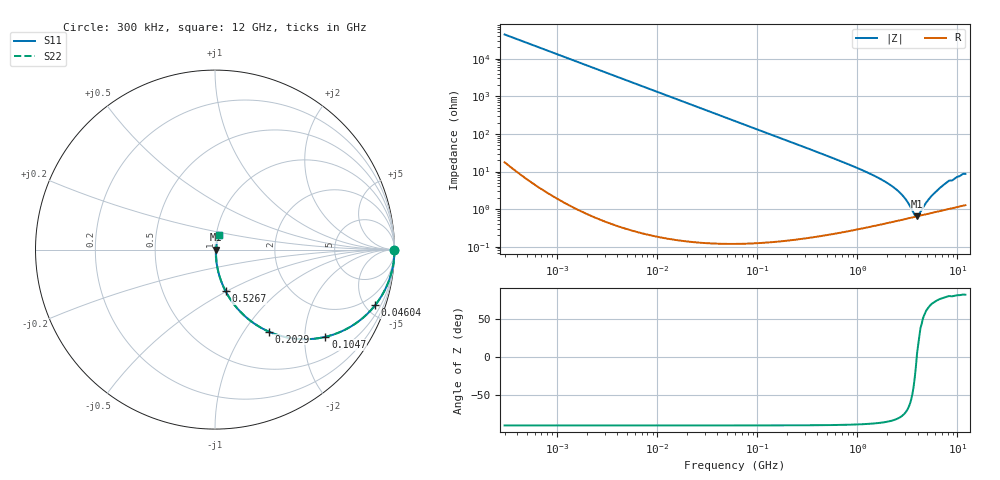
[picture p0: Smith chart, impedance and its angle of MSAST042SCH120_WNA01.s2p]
! MSAST042SCH120_WNA01  S-PARAMETER MODEL  ( General Type )
! Model Generated by TAIYO YUDEN Corporation (http://www.ty-top.com)
! Version 1.0
! TAIYO YUDEN Control No. 150820
! Copyright(c) 2015 TAIYO YUDEN CO.,LTD. All Rights Reserved.
! Product Description (link to TY-COMPAS)
! https://ds.yuden.co.jp/TYCOMPAS/or/detail?pn=MSAST042SCH120JWNA01&u=M
! Products Name : Multilayer Ceramic Capacitors
! Characteristics :
!  Capacitance : 12 pF , Rated Voltage : 25V , TCC : CH / C0H
!  Case Size : 0.4 x 0.2 / 0.016 x 0.008 [mm/inch] , Thickness : 0.2 / 0.008 [mm/inch]
!  (Conditions: Temperature = 25 degC , DC Bias Current/Voltage = 0A / 0V)
! External Node Assignments :
!  1  o---| |---o  2
! GND o---------o GND
! Frequency Range : 0.3MHz  -  12000MHz  [ 401 STEP ]
# MHz S RI R 50
! Freq[MHz].  S11 Real  S11 Imag  S21 Real  S21 Imag  S12 Real  S12 Imag  S22 Real  S22 Imag
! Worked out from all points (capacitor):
!   401 points, 300 kHz to 12 GHz, reference 50 ohm
!   read as one part in series: C = 12 pF near 316.3 kHz
!   lowest |Z| = 642 mohm at 3.944 GHz (marker M1)
!   series resonance near 3.92 GHz, so ESL is about 140 pH
!   S11 on the Smith chart (normalised r, x): 300 kHz: open; 46.04 MHz: 1.00, -5.75; 104.7 MHz: 1.00, -2.53; 202.9 MHz: 1.00, -1.30; 526.7 MHz: 1.00, -0.49; 12 GHz: 1.03, +0.17
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0.3  1 -0.00226  6.03e-06 0.00226  6.03e-06 0.00226  1 -0.00226
1.769972  0.9998 -0.0134  0.00018 0.0134  0.00018 0.0134  0.9998 -0.0134
10.44266  0.9938 -0.0783  0.00619 0.0783  0.00619 0.0783  0.9938 -0.0783
22.51442  0.9719 -0.1652  0.0281 0.1652  0.0281 0.1652  0.9719 -0.1652
46.03623  0.8921 -0.31  0.1079 0.31  0.1079 0.31  0.8921 -0.31
60  0.8296 -0.3757  0.1704 0.3757  0.1704 0.3757  0.8296 -0.3757
104.6549  0.6153 -0.486  0.3847 0.486  0.3847 0.486  0.6153 -0.486
143.8206  0.4584 -0.4975  0.5416 0.4975  0.5416 0.4975  0.4584 -0.4975
202.9496  0.2981 -0.4563  0.7019 0.4563  0.7019 0.4563  0.2981 -0.4563
353.9943  0.1223 -0.3252  0.8777 0.3252  0.8777 0.3252  0.1223 -0.3252
526.7124  0.0592 -0.2319  0.9408 0.2319  0.9408 0.2319  0.0592 -0.2319
1229.528  0.0125 -0.0957  0.9875 0.0957  0.9875 0.0957  0.0125 -0.0957
2088.533  0.00638 -0.045  0.9936 0.045  0.9936 0.045  0.00638 -0.045
2795.104  0.0057 -0.0231  0.9943 0.0231  0.9943 0.0231  0.0057 -0.0231
3190.978  0.00579 -0.0139  0.9942 0.0139  0.9942 0.0139  0.00579 -0.0139
3740.715  0.00617 -0.00323  0.9938 0.00323  0.9938 0.00323  0.00617 -0.00323
3944.255  0.00637 0.000444  0.9936 -0.000444  0.9936 -0.000444  0.00637 0.000444
4158.869  0.00659 0.00324  0.9934 -0.00324  0.9934 -0.00324  0.00659 0.00324
5278.635  0.00794 0.0178  0.9921 -0.0178  0.9921 -0.0178  0.00794 0.0178
6879.757  0.0104 0.0372  0.9896 -0.0372  0.9896 -0.0372  0.0104 0.0372
8064.993  0.0127 0.0523  0.9873 -0.0523  0.9873 -0.0523  0.0127 0.0523
12000  0.0196 0.0832  0.9804 -0.0832  0.9804 -0.0832  0.0196 0.0832
